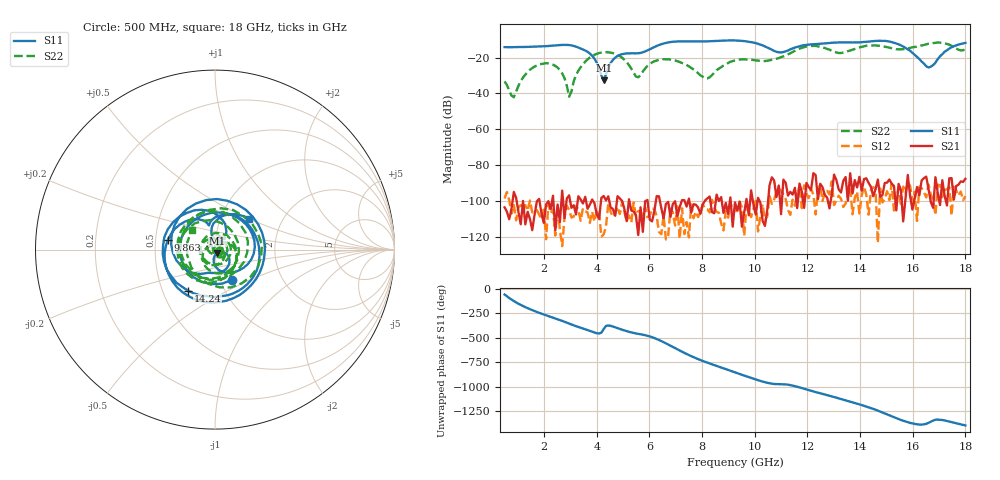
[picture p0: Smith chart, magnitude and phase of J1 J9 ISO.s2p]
!Agilent Technologies,N5230A,MY45001360,A.07.50.67
!Agilent N5230A: A.07.50.67
!Date: Tuesday, April 16, 2024 16:40:53
!Correction: S11(Full 2 Port(1,2))
!S21(Full 2 Port(1,2))
!S12(Full 2 Port(1,2))
!S22(Full 2 Port(1,2))
!S2P File: Measurements: S11, S21, S12, S22:
# Hz S  dB  R 50
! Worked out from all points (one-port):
!   201 points, 500 MHz to 18 GHz, reference 50 ohm
!   lowest |S11| = -32.7 dB at 4.263 GHz (marker M1), VSWR 1.05, Z = 51.4 - j1.9 ohm
!   |S11| at or under -10 dB: start of sweep to end of sweep
!   S11 on the Smith chart (normalised r, x): 500 MHz: 1.14, -0.40; 9.863 GHz: 0.58, +0.07; 14.24 GHz: 0.67, -0.33; 18 GHz: 1.35, +0.50
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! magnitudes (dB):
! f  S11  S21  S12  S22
! 500 MHz  -14.2  -103.4  -98.4  -33.3
! 850 MHz  -14.2  -94.8  -102.2  -42.1
! 1.462 GHz  -14.1  -109.9  -99.6  -26.8
! 2.25 GHz  -13.5  -104.3  -106.6  -23.6
! 2.688 GHz  -13.0  -94.1  -125.0  -28.9
! 2.95 GHz  -13.1  -96.7  -104.7  -41.8
! 3.475 GHz  -15.5  -101.3  -104.0  -23.8
! 3.913 GHz  -20.7  -101.1  -111.3  -18.5
! 4.263 GHz  -32.7  -97.1  -118.5  -17.1
! 4.7 GHz  -20.1  -108.1  -106.8  -18.0
! 5.575 GHz  -17.6  -118.8  -105.5  -31.0
! 6.362 GHz  -13.0  -97.3  -117.1  -21.3
! 8.2 GHz  -11.0  -98.4  -104.5  -31.6
! 9.25 GHz  -10.5  -100.6  -105.1  -21.6
! 9.863 GHz  -11.4  -94.0  -108.8  -21.2
! 11 GHz  -17.2  -107.2  -94.2  -19.7
! 12.22 GHz  -12.6  -84.4  -96.3  -13.5
! 13.28 GHz  -11.6  -95.1  -98.6  -17.5
! 14.24 GHz  -11.2  -87.2  -96.4  -13.4
! 15.11 GHz  -11.1  -87.9  -99.4  -14.5
! 16.6 GHz  -25.6  -93.2  -90.8  -12.3
! 18 GHz  -11.9  -87.5  -97.2  -15.4
